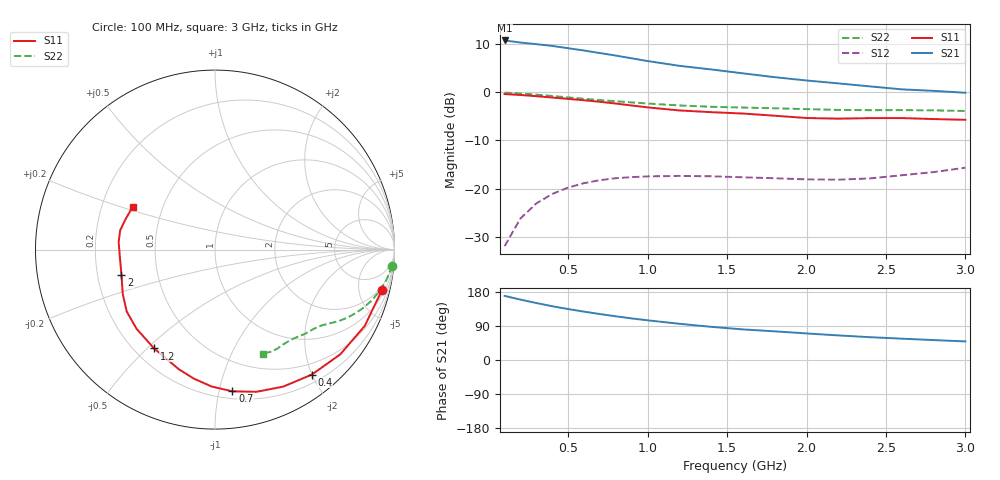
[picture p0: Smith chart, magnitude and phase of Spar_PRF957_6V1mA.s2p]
! Filename:  PRF957K.S2P  Version:  3.0
! NXP part #:  PRF957  Date:  Nov 1998
! Bias condition:  Vce=6V, Ic=1.0mA
#  MHz  S  MA  R 50
! Freq  S11  S21  S12  S22
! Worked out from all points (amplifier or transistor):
!   20 points, 100 MHz to 3 GHz, reference 50 ohm
!   highest |S21| = 10.7 dB at 100 MHz (marker M1)
!   |S21| within 3 dB of that: start of sweep to 773.7 MHz
!   unconditionally stable (mu >= 1): 2.052 GHz to end of sweep
!   at 400 MHz: K = 0.15, MSG = 15.4 dB, |S12| = -21.1 dB
!   at 1.2 GHz: K = 0.50, MSG = 11.4 dB, |S12| = -17.4 dB
!   at 3 GHz: K = 1.15, MAG = 5.4 dB, |S12| = -15.7 dB
!   lowest NFmin = 0.94 dB at 500 MHz
!   S11 on the Smith chart (normalised r, x): 100 MHz: 1.48, -8.02; 400 MHz: 0.32, -2.00; 700 MHz: 0.26, -1.10; 1.2 GHz: 0.28, -0.53; 2 GHz: 0.30, -0.12; 3 GHz: 0.34, +0.22
100  0.9569 -13.8  3.446 169.2  0.02524 81.6  0.991 -5.2
200  0.9363 -27.0  3.279 159.4  0.04902 74.2  0.9706 -10.0
300  0.9098 -39.9  3.154 150.3  0.07019 67.3  0.9441 -14.4
400  0.8809 -52.2  3.024 141.9  0.088 61.2  0.9143 -18.4
500  0.8529 -63.5  2.863 134.4  0.1024 56.2  0.8838 -21.9
600  0.8251 -73.8  2.709 127.5  0.1138 51.8  0.8547 -24.8
700  0.7954 -83.0  2.549 121.3  0.1223 48.1  0.8292 -27.2
800  0.7628 -91.5  2.402 115.3  0.1281 44.8  0.8058 -29.2
900  0.7283 -99.3  2.248 109.7  0.1315 42.3  0.7839 -30.9
1000  0.696 -106.9  2.106 104.8  0.1337 40.3  0.7635 -32.5
1200  0.6468 -121.6  1.879 95.6  0.1353 37.5  0.7287 -35.5
1400  0.6211 -134.7  1.724 87.5  0.1341 36.1  0.7062 -38.6
1600  0.6007 -145.0  1.57 80.7  0.131 37.2  0.6932 -41.6
1800  0.5703 -154.3  1.432 75.6  0.128 40.2  0.6817 -44.1
2000  0.5401 -164.8  1.324 70.1  0.1247 44.4  0.6679 -46.9
2200  0.5316 -175.7  1.235 64.9  0.1236 50.0  0.6556 -50.4
2400  0.5385 175.4  1.149 60.2  0.1275 56.5  0.6508 -54.4
2600  0.5391 168.5  1.071 56.3  0.1375 63.4  0.6522 -58.1
2800  0.5265 161.3  1.033 52.5  0.1483 69.9  0.6484 -61.4
3000  0.5171 152.7  0.9873 49.1  0.1648 75.3  0.6387 -65.2
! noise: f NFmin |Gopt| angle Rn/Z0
500  0.94  0.7  34  0.43
800  1.19  0.53  54  0.4
900  1.26  0.54  63  0.4
1000  1.5  0.53  70  0.38
1500  1.65  0.5  111  0.26
2000  2.09  0.53  166  0.08
